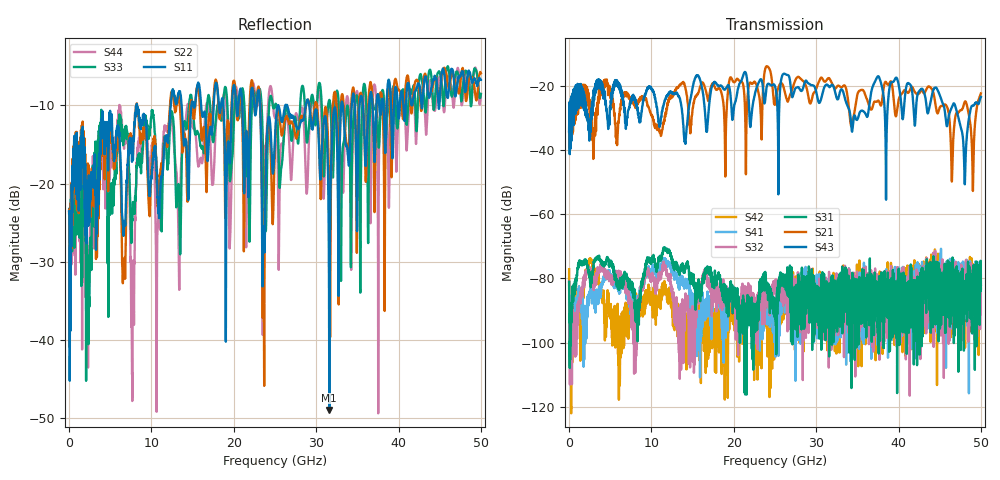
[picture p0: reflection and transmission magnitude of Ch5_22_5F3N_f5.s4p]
!Agilent Technologies,N5247A,US51170199,A.09.90.13
!Agilent N5247A: A.09.90.13
!Date: Wednesday, December 09, 2015 09:28:07
!Correction: S11(Full 4 Port(1,2,3,4))
!S12(Full 4 Port(1,2,3,4))
!S13(Full 4 Port(1,2,3,4))
!S14(Full 4 Port(1,2,3,4))
!S21(Full 4 Port(1,2,3,4))
!S22(Full 4 Port(1,2,3,4))
!S23(Full 4 Port(1,2,3,4))
!S24(Full 4 Port(1,2,3,4))
!S31(Full 4 Port(1,2,3,4))
!S32(Full 4 Port(1,2,3,4))
!S33(Full 4 Port(1,2,3,4))
!S34(Full 4 Port(1,2,3,4))
!S41(Full 4 Port(1,2,3,4))
!S42(Full 4 Port(1,2,3,4))
!S43(Full 4 Port(1,2,3,4))
!S44(Full 4 Port(1,2,3,4))
!S4P File: Measurements: <S11,S12,S13,S14>,
!<S21,S22,S23,S24>,
!<S31,S32,S33,S34>,
!<S41,S42,S43,S44>:
# Hz S  dB  R 50
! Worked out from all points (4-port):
!   3201 points, 10 MHz to 50 GHz, reference 50 ohm
!   strongest paths, dB at 10 MHz, 12.51 GHz, 25 GHz, 37.5 GHz, 50 GHz:
!     S43: -34.3, -22.4, -20.2, -17.1, -23.6
!     S21: -34.5, -23.5, -25.9, -24.7, -22.4
!     S31: -81.1, -74.2, -89.9, -88.8, -82.0
!     S32: -81.0, -83.7, -82.0, -86.1, -79.0
!     S41: -88.1, -78.4, -92.8, -90.8, -83.1
!     S42: -77.2, -87.4, -89.9, -91.8, -82.8
!   lowest |S11| = -49.0 dB at 31.6 GHz (marker M1), VSWR 1.01, Z = 50.2 - j0.257 ohm
!   |S11| at or under -10 dB: start of sweep to 8.216 GHz; 8.247 GHz to 12.35 GHz (4.099 GHz wide, 39.8 % of centre); 29.17 GHz to 33.04 GHz (3.873 GHz wide, 12.5 % of centre)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
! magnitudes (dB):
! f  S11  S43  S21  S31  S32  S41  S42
! 10 MHz  -23.8  -34.3  -34.5  -81.1  -81.0  -88.1  -77.2
! 7.712 GHz  -15.6  -23.3  -24.9  -84.5  -94.4  -87.9  -90.1
! 14.1 GHz  -14.6  -37.6  -20.3  -77.2  -89.7  -81.4  -95.6
! 15.68 GHz  -7.1  -16.9  -22.4  -83.9  -85.0  -98.1  -94.1
! 31.6 GHz  -49.0  -20.5  -17.7  -82.1  -81.7  -78.8  -91.1
! 48.05 GHz  -8.1  -50.7  -25.0  -86.8  -88.5  -83.7  -100.8
! 50 GHz  -6.7  -23.6  -22.4  -82.0  -79.0  -83.1  -82.8
